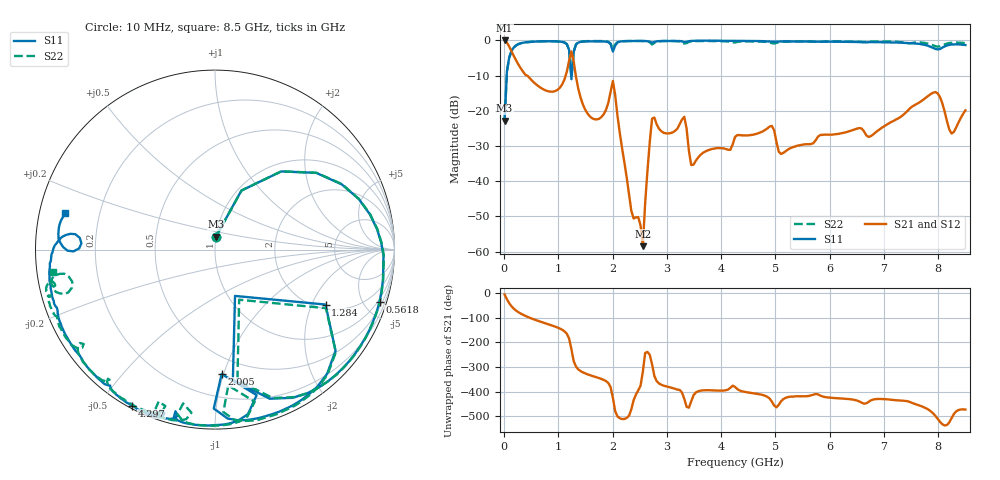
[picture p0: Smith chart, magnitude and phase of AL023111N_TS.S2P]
!AVX CORPORATION
!PN: AL023111N_TS
!DESCRIPTION: AIR CORE INDUCTOR, 111nH, 10 turns
!Agilent Technologies,E5071C,MY46102230,A.09.54
!Date: Mon Sep 03 16:44:08 2012
!Data & Calibration Information:
!Freq	S11:SOLT2(ON)	S21:SOLT2(ON)	S12:SOLT2(ON)	S22:SOLT2(ON)
# Hz S dB R 50
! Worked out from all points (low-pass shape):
!   201 points, 10 MHz to 8.5 GHz, reference 50 ohm
!   highest |S21| = -0.02 dB at 10 MHz (marker M1); lowest = -58.5 dB at 2.557 GHz (marker M2)
!   |S21| within 3 dB of the highest: start of sweep to 134.8 MHz
!   lowest |S11| = -22.8 dB at 10 MHz (marker M3), VSWR 1.16, Z = 50 + j7.27 ohm
!   |S11| at or under -10 dB: start of sweep to 49 MHz; 1.236 GHz to 1.247 GHz (10.8 MHz wide, 0.87 % of centre)
!   |S22| runs from -22.8 to -0.2 dB; largest |S21 - S12| = 0.011
!   S11 on the Smith chart (normalised r, x): 10 MHz: 1.00, +0.15; 561.9 MHz: 0.82, -6.35; 1.284 GHz: 2.18, -2.54; 2.005 GHz: 0.37, -0.98; 4.297 GHz: 0.01, -0.60; 8.5 GHz: 0.08, +0.12
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1e7  -22.80 85.6  -0.02 -4.7  -0.12 -4.7  -22.80 86.0
5.245e7  -8.87 65.9  -0.62 -24.0  -0.58 -24.1  -8.83 65.8
1.3735e8  -3.00 37.1  -3.10 -52.6  -3.09 -52.6  -2.98 37.1
5.6185e8  -0.34 -17.6  -12.12 -106.9  -12.12 -107.0  -0.32 -17.7
1.1986e9  -2.71 -82.2  -5.76 176.1  -5.76 176.0  -2.65 -80.2
1.24105e9  -11.02 -66.6  -3.11 132.3  -3.11 132.3  -10.17 -64.2
1.2835e9  -3.25 -26.4  -6.09 83.7  -6.08 83.6  -3.11 -27.8
1.4533e9  -0.34 -57.2  -18.24 38.2  -18.22 38.0  -0.29 -56.8
1.7929e9  -0.28 -77.2  -21.78 11.5  -21.80 11.5  -0.18 -76.0
2.00515e9  -3.17 -86.9  -11.52 -65.5  -11.52 -65.5  -2.38 -84.4
2.34475e9  -0.17 -92.1  -48.42 -112.4  -48.61 -112.9  -0.17 -90.7
2.557e9  -0.17 -99.2  -58.48 40.8  -58.67 42.9  -0.18 -97.6
2.7268e9  -0.65 -103.7  -22.23 71.0  -22.23 71.0  -1.16 -101.7
2.85415e9  -0.21 -105.1  -25.09 -6.8  -25.12 -6.9  -0.26 -101.4
3.3211e9  -0.48 -108.7  -21.72 -69.8  -21.73 -69.8  -0.89 -110.3
3.44845e9  -0.15 -108.2  -35.42 -79.7  -35.46 -79.8  -0.27 -109.7
4.255e9  -0.16 -117.6  -27.46 -20.8  -27.47 -20.7  -0.60 -129.0
4.29745e9  -0.14 -118.0  -26.90 -30.0  -26.88 -30.1  -0.43 -129.6
5.6983e9  -0.36 -140.9  -29.21 -52.7  -29.24 -52.8  -0.36 -156.4
7.09915e9  -0.55 -168.6  -23.49 -72.8  -23.51 -72.8  -0.30 -167.1
7.94815e9  -2.43 175.0  -14.68 -139.3  -14.69 -139.3  -1.64 -169.5
8.5e9  -1.31 166.4  -19.87 -113.3  -19.87 -113.2  -0.79 -172.3
